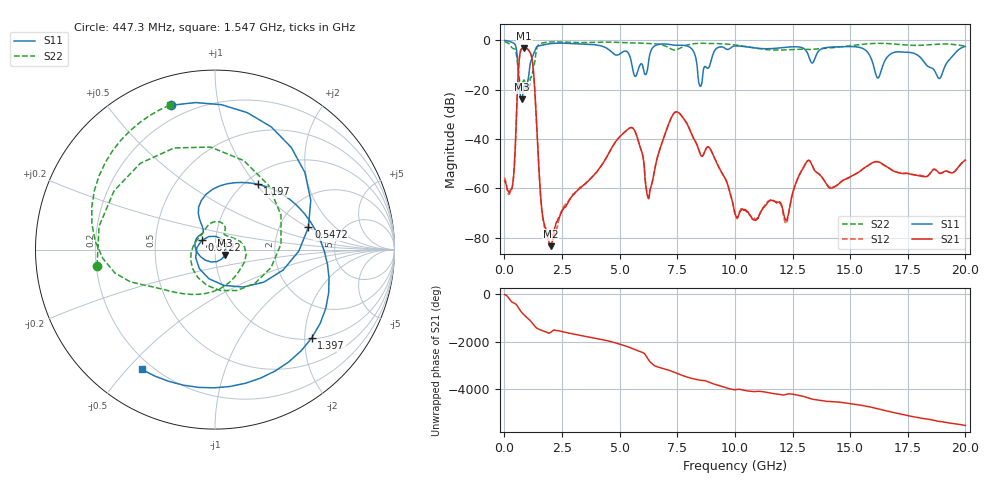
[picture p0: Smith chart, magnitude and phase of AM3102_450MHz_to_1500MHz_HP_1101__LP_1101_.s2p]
!Agilent Technologies,E8364B,MY43040894,A.07.50.67
!Agilent E8364B: A.07.50.67
!Date: Thursday, January 11, 2018 06:40:45
!Correction: S11(Full 2 Port(1,2))
!S21(Full 2 Port(1,2))
!S12(Full 2 Port(1,2))
!S22(Full 2 Port(1,2))
!S2P File: Measurements: S11, S21, S12, S22:
# Hz S  dB  R 50
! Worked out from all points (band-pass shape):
!   1601 points, 10 MHz to 20 GHz, reference 50 ohm
!   highest |S21| = -3.10 dB at 859.6 MHz (marker M1); lowest = -83.4 dB at 2.009 GHz (marker M2)
!   |S21| within 3 dB of the highest: 665.5 MHz to 1.166 GHz (500.1 MHz wide, 54.6 % of centre)
!   lowest |S11| = -23.9 dB at 747.1 MHz (marker M3), VSWR 1.14, Z = 55.9 - j3.28 ohm
!   |S11| at or under -10 dB: 586.6 MHz to 1.112 GHz (525.4 MHz wide, 61.9 % of centre); 8.357 GHz to 8.916 GHz (559.1 MHz wide, 6.47 % of centre); 18.31 GHz to 19.14 GHz (829 MHz wide, 4.43 % of centre)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
!   |S22| runs from -20.1 to -0.5 dB; largest |S21 - S12| = 0.0011
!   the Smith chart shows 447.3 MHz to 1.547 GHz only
!   S11 on the Smith chart (normalised r, x): 447.3 MHz: 0.13, +0.73; 547.2 MHz: 2.91, +1.01; 672.2 MHz: 0.86, +0.09; 1.197 GHz: 1.14, +1.02; 1.397 GHz: 1.03, -2.17; 1.547 GHz: 0.16, -0.55
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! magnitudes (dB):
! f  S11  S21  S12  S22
! 10 MHz  -0.1  -57.0  -55.6  -0.5
! 447.3 MHz  -1.5  -48.4  -48.6  -3.6
! 547.2 MHz  -5.4  -24.6  -24.6  -7.6
! 672.2 MHz  -21.0  -5.6  -5.6  -17.5
! 747.1 MHz  -23.9  -3.5  -3.5  -18.6
! 859.6 MHz  -18.4  -3.1  -3.1  -16.1
! 1.197 GHz  -7.2  -7.4  -7.4  -14.1
! 1.397 GHz  -2.7  -33.8  -33.8  -3.5
! 1.547 GHz  -2.1  -59.7  -59.6  -1.5
! 2.009 GHz  -1.3  -83.4  -78.4  -0.7
! 3.346 GHz  -1.5  -59.4  -59.2  -0.9
! 5.432 GHz  -6.2  -35.6  -35.6  -1.0
! 6.232 GHz  -10.4  -63.9  -63.2  -1.3
! 6.682 GHz  -1.7  -46.0  -46.0  -1.6
! 7.569 GHz  -2.0  -29.4  -29.4  -3.4
! 8.493 GHz  -18.6  -46.0  -46.0  -1.2
! 10.01 GHz  -2.3  -70.0  -70.5  -1.9
! 12.23 GHz  -2.8  -72.9  -74.3  -3.9
! 13.34 GHz  -9.2  -50.4  -50.4  -3.7
! 16.68 GHz  -6.1  -51.7  -51.7  -1.3
! 18.88 GHz  -15.5  -53.8  -53.8  -1.5
! 20 GHz  -2.5  -48.6  -48.4  -2.3
